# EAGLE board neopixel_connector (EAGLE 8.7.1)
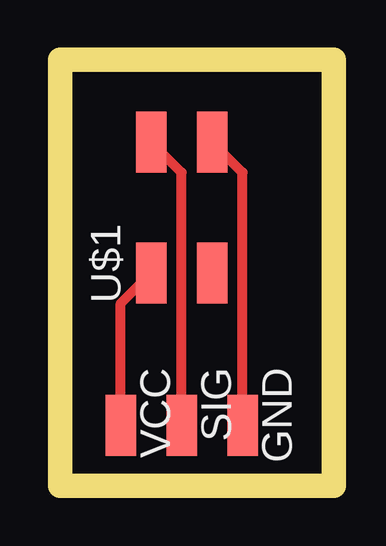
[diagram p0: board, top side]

Size 11.1 x 17.77 mm. Coordinates in mm from the lower left corner, seen from the top.
Outline: 0,0 11.1,0 11.1,17.77 0,17.77 0,0
Copper layers (1*16): Top 0.035mm / dielectric 1.5mm / Bottom 0.035mm
Design rules "default": minimum track width 6mil, minimum drill 0.35mm, track to track 6mil, track to pad 6mil, pad to pad 6mil, via to via 6mil, smd to smd 6mil, copper to edge 40mil, drill to drill 6mil, minimum pad ring 10mil, minimum via ring 8mil, stop-mask expansion 4mil, vias tented up to drill 0mil, thermal gap 10mil
Milling: 4 lines

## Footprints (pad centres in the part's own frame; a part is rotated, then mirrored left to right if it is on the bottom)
SMD1,27-2,54 = smd 1.27 x 2.54: 1 0,0
2X02SMD = smd 2.54 x 1.27: 1 -2.54,1.27; 2 2.92,1.27; 3 -2.54,-1.27; 4 2.92,-1.27

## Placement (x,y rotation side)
GND  [SMD1,27-2,54]  7.62,2.54 180 top
SIG  [SMD1,27-2,54]  5.08,2.54 180 top
U$1  [2X02SMD]  5.08,11.43 90 top
VCC  [SMD1,27-2,54]  2.54,2.54 180 top

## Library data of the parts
GND SIG VCC = wirepad
U$1 = fab

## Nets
N$1: U$1.1 VCC.1
N$2: SIG.1 U$1.2
N$3: GND.1 U$1.4

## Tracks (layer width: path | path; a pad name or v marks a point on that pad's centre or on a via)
N$1
  Top 0.406: VCC.1 2.54,7.62 U$1.1
N$2
  Top 0.406: SIG.1 5.08,13.08 U$1.2
N$3
  Top 0.406: GND.1 7.62,13.08 U$1.4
